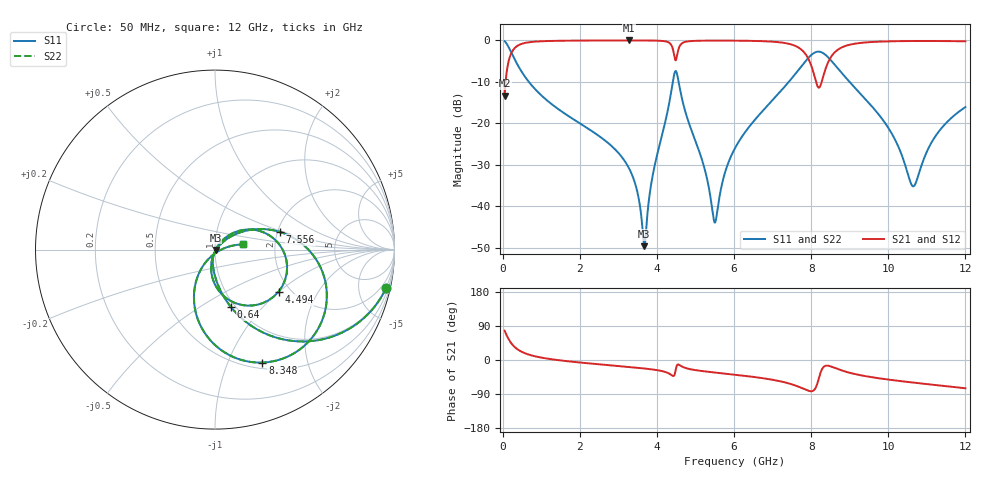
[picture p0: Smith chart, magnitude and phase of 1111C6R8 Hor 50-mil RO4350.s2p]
# GHz S MA R 50
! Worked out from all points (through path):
!   1601 points, 50 MHz to 12 GHz, reference 50 ohm
!   highest |S21| = -0.02 dB at 3.276 GHz (marker M1); lowest = -13.4 dB at 50 MHz (marker M2)
!   group delay of S21, straight-line fit = 19.3 ps
!   lowest |S11| = -49.7 dB at 3.672 GHz (marker M3), VSWR 1.01, Z = 50.3 - j0.172 ohm
!   |S11| at or under -10 dB: 676.9 MHz to 4.413 GHz (3.736 GHz wide, 147 % of centre); 4.563 GHz to 7.422 GHz (2.859 GHz wide, 47.7 % of centre); 8.994 GHz to end of sweep
!   |S22| runs from -49.7 to -0.2 dB; largest |S21 - S12| = 0
!   S11 on the Smith chart (normalised r, x): 50 MHz: 0.95, -8.90; 640 MHz: 0.95, -0.69; 4.494 GHz: 1.73, -0.99; 7.556 GHz: 2.07, +0.47; 8.348 GHz: 0.57, -1.34; 12 GHz: 1.36, +0.08
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0.05  0.9768 -12.7  0.2142 77.3  0.2142 77.3  0.9768 -12.7
0.2367188  0.6932 -47.6  0.7204 42.4  0.7204 42.4  0.6932 -47.6
0.6400313  0.3328 -74.4  0.9423 15.5  0.9423 15.5  0.3328 -74.4
2.044156  0.09675 -96.3  0.994 -7.1  0.994 -7.1  0.09675 -96.3
3.2765  0.02857 -104.3  0.9973 -18.4  0.9973 -18.4  0.02857 -104.3
3.672344  0.003284 -31.4  0.9965 -22.4  0.9965 -22.4  0.003284 -31.4
4.038312  0.04804 52.8  0.9904 -27.3  0.9904 -27.3  0.04804 52.8
4.366937  0.2343 28.4  0.886 -39.0  0.886 -39.0  0.2343 28.4
4.493906  0.4246 -33.5  0.5796 -22.6  0.5796 -22.6  0.4246 -33.5
4.688094  0.167 -93.9  0.9429 -19.1  0.9429 -19.1  0.167 -93.9
5.225844  0.02942 -104.9  0.9917 -29.8  0.9917 -29.8  0.02942 -104.9
5.494719  0.006353 -38.7  0.9934 -32.9  0.9934 -32.9  0.006353 -38.7
6.025  0.05001 43.6  0.9918 -38.8  0.9918 -38.8  0.05001 43.6
7.556094  0.3763 15.1  0.8699 -66.1  0.8699 -66.1  0.3763 15.1
8.019156  0.6752 -22.7  0.471 -82.3  0.471 -82.3  0.6752 -22.7
8.190938  0.7316 -46.0  0.2689 -51.6  0.2689 -51.6  0.7316 -46.0
8.347781  0.6827 -67.2  0.4167 -16.4  0.4167 -16.4  0.6827 -67.2
8.818312  0.3913 -104.7  0.8318 -28.4  0.8318 -28.4  0.3913 -104.7
10.01331  0.0861 -126.4  0.9731 -51.8  0.9731 -51.8  0.0861 -126.4
10.65563  0.01732 -53.5  0.9823 -59.7  0.9823 -59.7  0.01732 -53.5
11.21578  0.06892 11.5  0.9823 -66.0  0.9823 -66.0  0.06892 11.5
12  0.1568 10.6  0.9739 -74.6  0.9739 -74.6  0.1568 10.6
